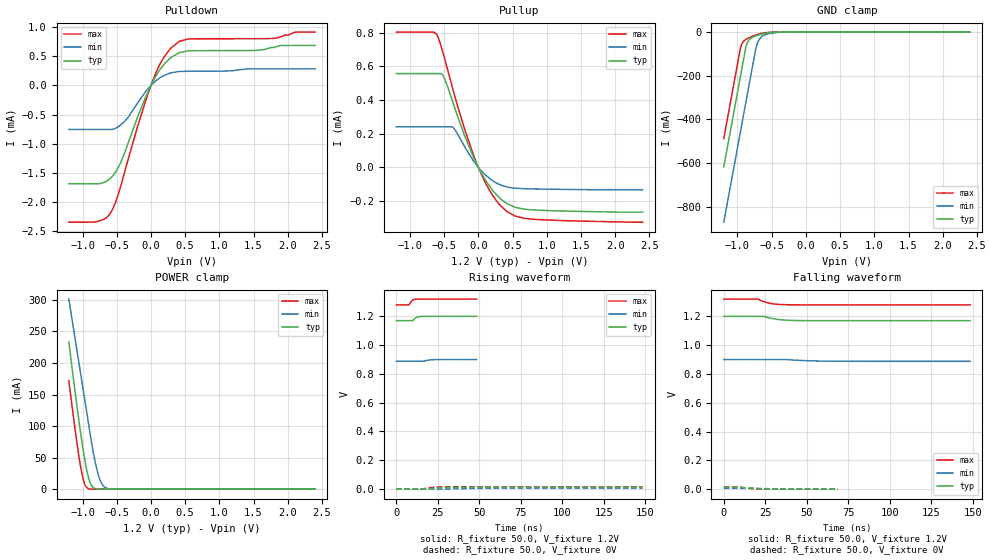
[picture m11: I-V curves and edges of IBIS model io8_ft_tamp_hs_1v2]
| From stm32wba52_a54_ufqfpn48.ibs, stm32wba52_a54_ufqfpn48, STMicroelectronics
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[Model]   io8_ft_tamp_hs_1v2
Model_type I/O
Polarity   Non-Inverting
Enable   Active-Low
| CAP_THRESHOLD on pad IOFT is "UDTCAPC" :
| Rising=30.0% of vddiom   Falling=70.0% of vddiom
| C_comp min and max val. don't necessarily correlate with the min and max pvt
| but are the smallest and greatest pad capacitance found.
| var   typ   min   max
C_comp   4.69898pF  4.28274pF  4.82428pF
|C_comp_pullup   2.96111pF  2.69812pF  2.96563pF
|C_comp_pulldown   1.73787pF  1.58461pF  1.85865pF
Vinl = 450.0mV
Vinh = 660.0mV
Vmeas = 600.0mV   | Reference voltage for timing measurements
Cref  = 50.0pF   | Timing specification test load capacitance value
Rref  = 1.0MOhm   | Timing specification test load resistance value
Vref  = 660.0mV   | Timing specification test load voltage
[Model Spec]
| TIME_THRESHOLD on pin ZIV33SW is "CMOS" :
| Rising=50.0% of VDDV33SW   Falling=50.0% of VDDV33SW
Vinl 436.50000mV 342.50000mV 466.50000mV
Vinh 753.50000mV 549.50000mV 839.50000mV
| variable   typ   min   max
[Temperature Range] 25.0 140.0 -40.0
| variable   typ   min   max
[Voltage Range] 1.2V 900.0mV 1.32V
| variable   typ   min   max
[POWER Clamp Reference] 1.2V 900.0mV 1.32V
| variable   typ   min   max
[GND Clamp Reference] 0V 0V 0V
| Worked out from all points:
|   slope of the pulldown table from 0 to 0.18 V, typ, clamps not added: 517 ohm
|   slope of the pullup table from 0 to 0.18 V, typ, clamps not added: 1.49 kohm
|   GND clamp passes 1 mA (typ) near -0.47 V on its own axis
|   POWER clamp passes 1 mA (typ) near -0.81 V on its own axis
[POWER Clamp]
-1.2V     233.4mA    301.3mA    171.8mA
-1.06V    114.5mA    205.3mA    57.35mA
-1.02V    83.5mA     177.8mA    30.99mA
-980mV    55.21mA    150.4mA    11.87mA
-920mV    21.5mA     109.2mA    1.195mA
-870mV    6.13mA     75.36mA    121.6uA
-820mV    1.189mA    45.7mA     11.82uA
-770mV    199.4uA    22.94mA    1.144uA
-730mV    46.68uA    11.1mA     176.6nA
-680mV    7.557uA    3.666mA    17.16nA
-510mV    15.46nA    46.13uA    134.2pA
2.4V      0A         0A         0A
[GND Clamp]
-1.2V     -616.6mA   -870.4mA   -486.7mA
-960mV    -208.6mA   -462.4mA   -78.75mA
-940mV    -174.6mA   -428.4mA   -56.97mA
-880mV    -73.49mA   -326.4mA   -34.53mA
-850mV    -45.28mA   -275.4mA   -29.09mA
-810mV    -29.66mA   -207.4mA   -23mA
-730mV    -17.09mA   -73.72mA   -13.06mA
-690mV    -13mA      -37.99mA   -9.157mA
-640mV    -8.81mA    -19.57mA   -5.341mA
-520mV    -2.385mA   -6.292mA   -748.7uA
-300mV    -8.501uA   -273.8uA   -150.7nA
2.4V      1.845nA    2.377uA    739.2pA
| variable   typ   min   max
[Pullup Reference] 1.2V 900.0mV 1.32V
| variable   typ   min   max
[Pulldown Reference] 0V 0V 0V
[Pullup]
-1.2V     556.9uA    241.1uA    803uA
-650mV    556.9uA    241.1uA    803uA
-610mV    556.9uA    241.1uA    789uA
-510mV    539.1uA    241.1uA    669.2uA
-370mV    382.5uA    236.9uA    459uA
-200mV    186.4uA    122.2uA    224.9uA
-30mV     24.45uA    15.08uA    29.88uA
190mV     -126.1uA   -73.56uA   -154.1uA
420mV     -215.5uA   -116.6uA   -262.7uA
540mV     -237.4uA   -123.5uA   -289.1uA
790mV     -252uA     -127.5uA   -307.1uA
2.4V      -265.4uA   -132.2uA   -325uA
[Pulldown]
-1.2V     -1.691mA   -757.3uA   -2.353mA
-760mV    -1.691mA   -757.3uA   -2.334mA
-580mV    -1.582mA   -757.3uA   -2.173mA
-430mV    -1.293mA   -666.6uA   -1.684mA
-200mV    -558.4uA   -310.3uA   -726.5uA
10mV      24.06uA    11.99uA    32.4uA
150mV     302.2uA    144.8uA    405.5uA
290mV     480.2uA    217.4uA    644uA
540mV     595.8uA    244.2uA    798.9uA
1.76V     653.9uA    285.4uA    807.9uA
2.11V     688.3uA    285.4uA    916.9uA
2.4V      688.3uA    285.4uA    918.5uA
[Ramp]
dV/dt_r 7.74246mV/8.41956ns 3.84635mV/15.25626ns 9.49142mV/6.51731ns
dV/dt_f 18.01416mV/8.8158ns 7.34518mV/14.8485ns 24.13953mV/7.2801ns
R_load = 50.0
| Removed startup time: 0s 0s 0s  .
| Removed end time: 48.4ns.
[Rising Waveform]
R_fixture   = 50.0
V_fixture   = 1.2V
V_fixture_min = 900.0mV
V_fixture_max = 1.32V
0s        1.17V      887.8mV    1.28V
7.55ns    1.17V      887.8mV    1.28V
8ns       1.17V      887.8mV    1.284V
9.8ns     1.17V      887.8mV    1.312V
11.85ns   1.191V     887.8mV    1.319V
13.85ns   1.198V     887.8mV    1.32V
15.8ns    1.2V       887.8mV    1.32V
19.75ns   1.2V       896.4mV    1.32V
22.75ns   1.2V       899.1mV    1.32V
48.4ns    1.2V       900mV      1.32V
| Removed startup time: 0s 0s 0s  .
| Removed end time: 148.4ns.
[Falling Waveform]
R_fixture   = 50.0
V_fixture   = 1.2V
V_fixture_min = 900.0mV
V_fixture_max = 1.32V
0s        1.2V       900mV      1.32V
20.85ns   1.2V       900.1mV    1.319V
21.8ns    1.2V       900mV      1.312V
24.25ns   1.2V       900mV      1.302V
27.95ns   1.188V     900mV      1.29V
31.6ns    1.18V      900mV      1.284V
37.15ns   1.174V     899.9mV    1.281V
51.5ns    1.17V      891.5mV    1.28V
64.15ns   1.17V      888.7mV    1.28V
148.4ns   1.17V      887.8mV    1.28V
| Removed startup time: 0s 0s 0s  .
| Removed end time: 148.4ns.
[Rising Waveform]
R_fixture   = 50.0
V_fixture   = 0V
V_fixture_min = 0V
V_fixture_max = 0V
0s        19.98nV    4.257uV    19.22nV
9.35ns    16.72uV    4.248uV    -800uV
15.15ns   -318.2uV   16.45uV    131.2uV
18.25ns   45.28uV    -309.2uV   5.69mV
22ns      4.039mV    -227.6uV   11.33mV
26.05ns   8.146mV    -36.01uV   14.38mV
30.2ns    10.79mV    164.6uV    15.46mV
37.05ns   12.51mV    1.901mV    15.81mV
58.9ns    12.91mV    5.965mV    15.82mV
148.4ns   12.9mV     6.415mV    15.82mV
| Removed startup time: 0s 0s 0s  .
| Removed end time: 68.4ns.
[Falling Waveform]
R_fixture   = 50.0
V_fixture   = 0V
V_fixture_min = 0V
V_fixture_max = 0V
0s        12.91mV    6.42mV     15.82mV
8.15ns    12.91mV    6.42mV     15.82mV
11.1ns    12.63mV    6.42mV     11.19mV
15.85ns   7.099mV    6.418mV    4.412mV
18.25ns   4.734mV    6.436mV    2.076mV
20.95ns   2.513mV    5.508mV    830.9uV
23.75ns   1.011mV    4.372mV    271.4uV
27.95ns   286.3uV    2.859mV    112.8uV
37.7ns    42.32uV    586uV      11.67uV
68.4ns    -262.7nV   14.68uV    24.39nV
